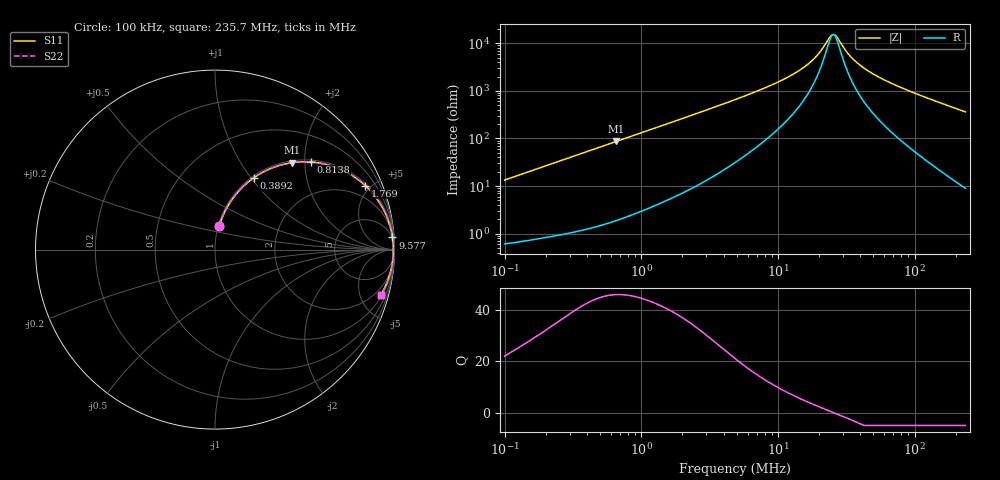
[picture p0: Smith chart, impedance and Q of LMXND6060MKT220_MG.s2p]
! LMXND6060MKT220_MG  S-PARAMETER MODEL  ( General Type )
! Model Generated by TAIYO YUDEN Corporation (https://www.yuden.co.jp/en/)
! Version 1.0
! TAIYO YUDEN Control No. 191025NI43SB-FBB
! Copyright(c) 2019 TAIYO YUDEN CO.,LTD. All Rights Reserved.
! Product Description (link to TY-COMPAS)
! https://ds.yuden.co.jp/TYCOMPAS/or/detail?pn=LMXND6060MKT220MMG&u=M
! Products Name : Inductors
! Characteristics :
!  Inductance : 22 uH , SRF(min) : 12 MHz , DC Resistance(max) : 0.558 Ohm
!  Rated Current : Saturation :760 mA , Temp Rise : 650 mA (40 degC)
!  Case Size : 6.0 x 6.0 / 0.236 x 0.236 [mm/inch] , Thickness : 1.2 / 0.047 [mm/inch]
!  (Conditions: Temperature = 25 degC , DC Bias Current/Voltage = 0A / 0V)
! External Node Assignments :
!  1  o---GGG---o  2
! GND o---------o GND
! Frequency Range : 0.1MHz  -  235.669543MHz  [ 402 STEP ]
# MHz S RI R 50
! Freq[MHz].  S11 Real  S11 Imag  S21 Real  S21 Imag  S12 Real  S12 Imag  S22 Real  S22 Imag
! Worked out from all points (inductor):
!   401 points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, 100 kHz to 235.7 MHz, reference 50 ohm
!   read as one part in series: L = 21.2 uH near 104 kHz
!   highest Q = 45.8 at 657.3 kHz (marker M1), where L = 20.9 uH
!   self-resonance near 25.28 MHz
!   S11 on the Smith chart (normalised r, x): 100 kHz: 1.01, +0.27; 389.2 kHz: 1.02, +1.03; 813.8 kHz: 1.05, +2.14; 1.769 MHz: 1.12, +4.64; 9.577 MHz: 4, +29; 235.7 MHz: 1.18, -7.23
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0.1  0.0233 0.1298  0.9767 -0.1298  0.9767 -0.1298  0.0233 0.1298
0.209107  0.0783 0.2537  0.9217 -0.2537  0.9217 -0.2537  0.0783 0.2537
0.367165  0.1963 0.3853  0.8037 -0.3853  0.8037 -0.3853  0.1963 0.3853
0.389182  0.2146 0.3988  0.7854 -0.3988  0.7854 -0.3988  0.2146 0.3988
0.65733  0.4297 0.4842  0.5703 -0.4842  0.5703 -0.4842  0.4297 0.4842
0.813808  0.533 0.488  0.467 -0.488  0.467 -0.488  0.533 0.488
1.348099  0.7525 0.4198  0.2475 -0.4198  0.2475 -0.4198  0.7525 0.4198
1.7691  0.837 0.3566  0.163 -0.3566  0.163 -0.3566  0.837 0.3566
2.764775  0.923 0.2511  0.077 -0.2511  0.077 -0.2511  0.923 0.2511
4.854581  0.9705 0.1471  0.0295 -0.1471  0.0295 -0.1471  0.9705 0.1471
9.576973  0.9887 0.0678  0.0113 -0.0678  0.0113 -0.0678  0.9887 0.0678
13.84882  0.992 0.0386  0.00804 -0.0386  0.00804 -0.0386  0.992 0.0386
17.8243  0.993 0.0217  0.00698 -0.0217  0.00698 -0.0217  0.993 0.0217
20.41869  0.9933 0.0133  0.00667 -0.0133  0.00667 -0.0133  0.9933 0.0133
24.3167  0.9935 0.00275  0.00649 -0.00275  0.00649 -0.00275  0.9935 0.00275
25.7749  0.9935 -0.000729  0.00648 0.000729  0.00648 0.000729  0.9935 -0.000729
27.32054  0.9935 -0.00421  0.00649 0.00421  0.00649 0.00421  0.9935 -0.00421
32.53614  0.9933 -0.0148  0.00669 0.0148  0.00669 0.0148  0.9933 -0.0148
38.0025  0.9929 -0.0245  0.00707 0.0245  0.00707 0.0245  0.9929 -0.0245
47.97127  0.9919 -0.0403  0.00811 0.0403  0.00811 0.0403  0.9919 -0.0403
65.44454  0.9893 -0.0648  0.0107 0.0648  0.0107 0.0648  0.9893 -0.0648
235.6695  0.9235 -0.2537  0.0765 0.2537  0.0765 0.2537  0.9235 -0.2537
